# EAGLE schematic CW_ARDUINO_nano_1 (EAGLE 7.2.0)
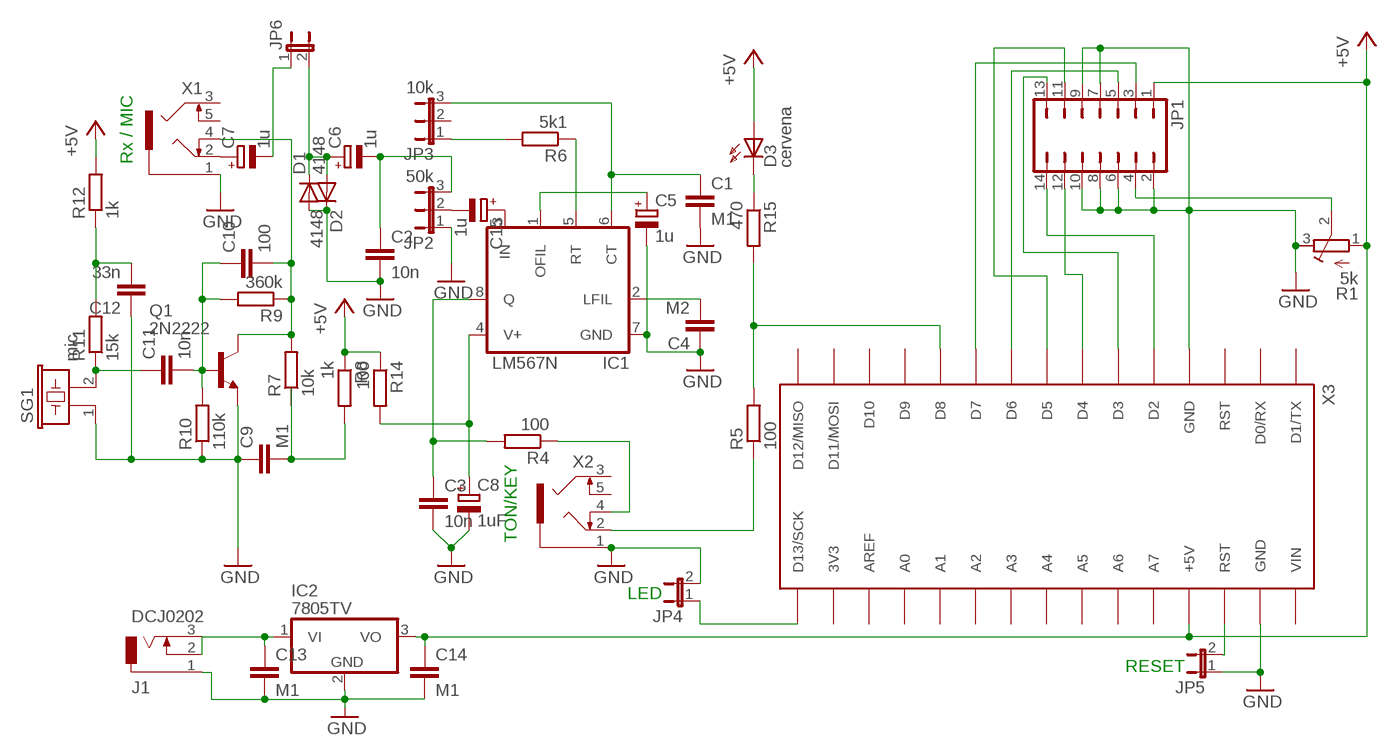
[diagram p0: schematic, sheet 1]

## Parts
C1  M1  C-EU050-030X075  [C050-030X075]
C2  10n  C-EU050-030X075  [C050-030X075]
C3  10n  C-EU050-030X075  [C050-030X075]
C4  M2  C-EU050-030X075  [C050-030X075]
C5  1u  CPOL-EUE2.5-5  [E2,5-5]
C6  1u  CPOL-EUE2.5-5  [E2,5-5]
C7  1u  CPOL-EUE2.5-5  [E2,5-5]
C8  1uF  CPOL-EUE2.5-5  [E2,5-5]
C9  M1  C-EU050-030X075  [C050-030X075]
C10  100  C-EU050-030X075  [C050-030X075]
C11  10n  C-EU050-030X075  [C050-030X075]
C12  33n  C-EU050-030X075  [C050-030X075]
C13  M1  C-EU050-030X075  [C050-030X075]
C14  M1  C-EU050-030X075  [C050-030X075]
C15  1u  CPOL-EUE2.5-5  [E2,5-5]
D1  4148  1N4148DO35-7  [DO35-7]
D2  4148  1N4148DO35-7  [DO35-7]
D3  cervena  HLMP6  [HLMP6]
IC1  LM567N  [DIL08]
IC2  7805TV  [TO220V]
J1  DCJ0202  [DCJ0202]
JP1  JP7Q  [JP7Q]
JP2  50k  JP2E  [JP2]
JP3  10k  JP2E  [JP2]
JP4  JP1E  [JP1]
JP5  JP1E  [JP1]
JP6  JP1E  [JP1]
Q1  2N2222  [TO18]
R1  5k  R-TRIMM3296P  [RTRIM3296P]
R4  100  R-EU_0207/10  [0207/10]
R5  100  R-EU_0207/10  [0207/10]
R6  5k1  R-EU_0207/10  [0207/10]
R7  10k  R-EU_0207/10  [0207/10]
R8  1k  R-EU_0207/10  [0207/10]
R9  360k  R-EU_0207/10  [0207/10]
R10  110k  R-EU_0207/10  [0207/10]
R11  15k  R-EU_0207/10  [0207/10]
R12  1k  R-EU_0207/10  [0207/10]
R14  100  R-EU_0207/10  [0207/10]
R15  470  R-EU_0207/10  [0207/10]
SG1  mic  EFBAA40D101  [EFBAA40D101]
X1  1503_09  [1503_09]
X2  1503_09  [1503_09]
X3  ARDUINO_NANO_COM  [ARDUINO_NANO_C]

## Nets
+5V: C14.1 D3.A IC2.3(VO) JP1.1 R1.1(A) R8.1 R12.2 R14.1 X3.27(+5V)
GND: C1.2 C2.2 C3.2 C4.1 C5.- C8.- C9.1 C12.1 C13.2 C14.2 D1.A D2.C IC1.7(GND) IC2.2(GND) J1.1 JP1.2 JP1.6 JP1.8 JP1.10 JP2.1 JP4.2 JP5.1 Q1.1(E) R1.3(E) R10.1 SG1.1 X1.1 X2.1 X3.4(GND) X3.29(GND)
N$2: JP1.4 R1.2(S)
N$3: JP4.1 X3.16(D13/SCK)
N$4: JP1.3 X3.10(D7)
N$5: C15.+ IC1.3(IN)
N$6: JP1.5 X3.9(D6)
N$7: C8.+ IC1.4(V+) R14.2
N$8: R4.1 X2.4
N$9: D3.K R15.1
N$10: JP3.1 R6.2
N$11: IC1.5(RT) R6.1
N$12: C1.1 IC1.6(CT) JP3.3
N$13: C3.1 IC1.8(Q) R4.2
N$14: R5.1 X2.2
N$15: C4.2 IC1.2(LFIL)
N$16: JP1.14 X3.5(D2)
N$17: C5.+ IC1.1(OFIL)
N$18: JP1.12 X3.7(D4)
N$19: R5.2 R15.2 X3.11(D8)
N$20: C2.1 C6.- JP2.3
N$21: JP1.13 X3.6(D3)
N$22: JP1.11 X3.8(D5)
N$23: C6.+ D1.C D2.A JP6.2
N$24: C10.2 Q1.3(C) R7.2 R9.1 X1.4
N$25: C7.+ X1.2
N$26: C9.2 R7.1 R8.2
N$27: C10.1 C11.2 Q1.2(B) R9.2 R10.2
N$28: C12.2 R11.2 R12.1
N$29: C11.1 R11.1 SG1.2
N$30: JP5.2 X3.28(RST)
N$31: C15.- JP2.2
N$32: C7.- JP6.1
N$33: C13.1 IC2.1(VI) J1.2 J1.3
Unconnected: JP1.7 JP1.9 JP3.2 X1.3 X1.5 X2.3 X2.5 X3.1(D1/TX) X3.2(D0/RX) X3.3(RST) X3.12(D9) X3.13(D10) X3.14(D11/MOSI) X3.15(D12/MISO) X3.17(3V3) X3.18(AREF) X3.19(A0) X3.20(A1) X3.21(A2) X3.22(A3) X3.23(A4) X3.24(A5) X3.25(A6) X3.26(A7) X3.30(VIN)

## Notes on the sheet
- Rx / MIC
- TON/KEY
- LED
- RESET

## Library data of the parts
C1-C4 C9-C14 = rcl:C-EU: CAPACITOR, European symbol
C5-C8 C15 = rcl:CPOL-EU: POLARIZED CAPACITOR, European symbol
D1 D2 = diode:1N4148: DIODE
D3 = display-hp:HLMP6: LED; MF: AGILENT TECHNOLOGIES; MPN: HLMP-6500; OC_FARNELL: 1652490; OC_NEWARK: 40K0088
IC1 = linear:*567: TONE DECODER
IC2 = linear:78*: Positive VOLTAGE REGULATOR Source: http://cache.national.com/ds/LM/LM78L05.pdf http://www.fairchildsemi.com/ds/LM/LM7805.pdf
J1 = con-jack:DCJ0202: DC POWER JACK Source: DCJ0202.pdf; OC_FARNELL: unknown; OC_NEWARK: unknown
JP1 = jumper:JP7Q: JUMPER
JP2 JP3 = jumper:JP2E: JUMPER
JP4-JP6 = jumper:JP1E: JUMPER
Q1 = transistor-npn:2N2222*: NPN Transistor
R1 = rcl:R-TRIMM: Trimm resistor
R4-R12 R14 R15 = rcl:R-EU_: RESISTOR, European symbol
SG1 = buzzer:EFB?: Piezoelectric Acoustic Transducer; OC_FARNELL: unknown; OC_NEWARK: unknown
X1 X2 = con-lumberg:1503_09: Jack connectors according to JISC 6560, 3.5 mm Klinkeneinbaukupplung nach JISC 6560, 3,5 mm, 3-polig/ stereo, abgewinkelte Ausführung, mit 2 Öffnern und Lötaugen, für Leiterplatten Rückseitenmontage Source: http://www.lumberg.com/Produkte/PDFs/1503_09.pdf; OC_FARNELL: 1243244; OC_NEWARK: unknown
X3 = Arduino_FB:ARDUINO_NANO_COM: Arduino Nano V3.0 Footprint as component for own designs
